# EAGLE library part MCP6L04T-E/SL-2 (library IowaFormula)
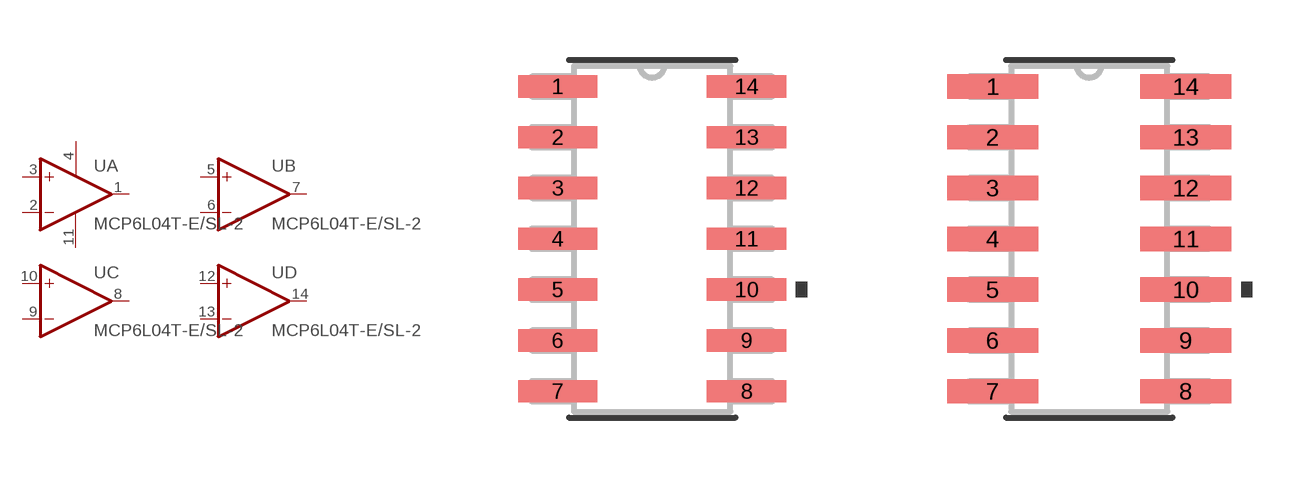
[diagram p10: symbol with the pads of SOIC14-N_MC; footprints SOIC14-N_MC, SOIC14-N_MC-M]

Designator prefix U; gates A=OPAMP B=OPAMP C=OPAMP D=OPAMP E=PWR+-

## MCP6L04T-E/SL-2 (MANUFACTURER_PART_NUMBER: MCP6L04TESL; VENDOR: Microchip)  [SOIC14-N_MC]
1  A:OUT  out
2  A:-IN  in
3  A:+IN  in
4  E:V+  pwr
5  B:+IN  in
6  B:-IN  in
7  B:OUT  out
8  C:OUT  out
9  C:-IN  in
10  C:+IN  in
11  E:V-  pwr
12  D:+IN  in
13  D:-IN  in
14  D:OUT  out

## MCP6L04T-E/SL-2SOIC14-N_MC-M (MANUFACTURER_PART_NUMBER: MCP6L04TESL; VENDOR: Microchip)  [SOIC14-N_MC-M]
Pads as for SOIC14-N_MC

## MCP6L04T-E/SL-2SOIC14-N_MC-L (MANUFACTURER_PART_NUMBER: MCP6L04TESL; VENDOR: Microchip)  [SOIC14-N_MC-L]
Pads as for SOIC14-N_MC

## Footprint SOIC14-N_MC (pad centres in mm)
smd 1.981 x 0.559: 1 -2.362,3.81; 2 -2.362,2.54; 3 -2.362,1.27; 4 -2.362,0; 5 -2.362,-1.27; 6 -2.362,-2.54; 7 -2.362,-3.81; 8 2.362,-3.81; 9 2.362,-2.54; 10 2.362,-1.27; 11 2.362,0; 12 2.362,1.27; 13 2.362,2.54; 14 2.362,3.81

## Footprint SOIC14-N_MC-M (pad centres in mm)
smd 2.286 x 0.61: 1 -2.413,3.81; 2 -2.413,2.54; 3 -2.413,1.27; 4 -2.413,0; 5 -2.413,-1.27; 6 -2.413,-2.54; 7 -2.413,-3.81; 8 2.413,-3.81; 9 2.413,-2.54; 10 2.413,-1.27; 11 2.413,0; 12 2.413,1.27; 13 2.413,2.54; 14 2.413,3.81

## Footprint SOIC14-N_MC-L (pad centres in mm)
smd 1.676 x 0.508: 1 -2.311,3.81; 2 -2.311,2.54; 3 -2.311,1.27; 4 -2.311,0; 5 -2.311,-1.27; 6 -2.311,-2.54; 7 -2.311,-3.81; 8 2.311,-3.81; 9 2.311,-2.54; 10 2.311,-1.27; 11 2.311,0; 12 2.311,1.27; 13 2.311,2.54; 14 2.311,3.81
